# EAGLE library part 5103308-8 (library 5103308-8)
HEADER, 2.54MM, 40WAY
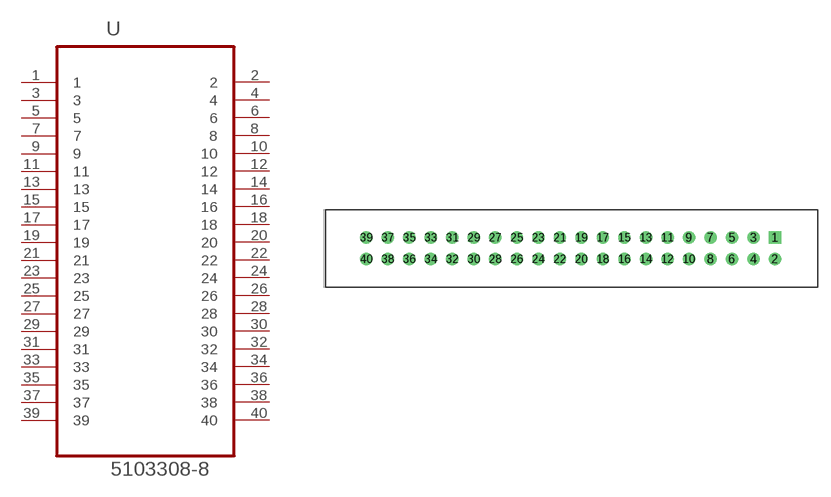
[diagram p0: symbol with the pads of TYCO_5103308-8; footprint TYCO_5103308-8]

Designator prefix U

## 5103308-8 (Centerline_Pitch: 2.54 mm[.1 in]; Comment: 5103308-8; Description: A/L LOW PRO HDR 40P VERT BLACK; Digi-Key_Part_Number: A33170-ND; Digi-Key_Purchase_URL: https://www.digikey.com/product-detail/en/te-connectivity-amp-connectors/5103308-8/A33170-ND/1114908?utm_source=snapeda&utm_medium=aggregator&utm_campaign=symbol; EU_RoHS_Compliance: Compliant; MF: TE Connectivity; MP: 5103308-8; Number_of_Positions: 40; Package: None; Product_Type: Connector; TE_purchase_URL: https://www.te.com/usa-en/product-5103308-8.html?te_bu=Cor&te_type=disp&te_campaign=seda_glo_cor-seda-global-disp-prtnr-fy19-seda-model-bom-cta_sma-317_1&elqCampaignId=32493)  [TYCO_5103308-8]
1  1  pas
2  2  pas
3  3  pas
4  4  pas
5  5  pas
6  6  pas
7  7  pas
8  8  pas
9  9  pas
10  10  pas
11  11  pas
12  12  pas
13  13  pas
14  14  pas
15  15  pas
16  16  pas
17  17  pas
18  18  pas
19  19  pas
20  20  pas
21  21  pas
22  22  pas
23  23  pas
24  24  pas
25  25  pas
26  26  pas
27  27  pas
28  28  pas
29  29  pas
30  30  pas
31  31  pas
32  32  pas
33  33  pas
34  34  pas
35  35  pas
36  36  pas
37  37  pas
38  38  pas
39  39  pas
40  40  pas

## Footprint TYCO_5103308-8 (pad centres in mm)
drill 0.965 square: 1 0,2.54
drill 0.965: 2 0,0; 3 -2.54,2.54; 4 -2.54,0; 5 -5.08,2.54; 6 -5.08,0; 7 -7.62,2.54; 8 -7.62,0; 9 -10.16,2.54; 10 -10.16,0; 11 -12.7,2.54; 12 -12.7,0; 13 -15.24,2.54; 14 -15.24,0; 15 -17.78,2.54; 16 -17.78,0; 17 -20.32,2.54; 18 -20.32,0; 19 -22.86,2.54; 20 -22.86,0; 21 -25.4,2.54; 22 -25.4,0; 23 -27.94,2.54; 24 -27.94,0; 25 -30.48,2.54; 26 -30.48,0; 27 -33.02,2.54; 28 -33.02,0; 29 -35.56,2.54; 30 -35.56,0; 31 -38.1,2.54; 32 -38.1,0; 33 -40.64,2.54; 34 -40.64,0; 35 -43.18,2.54; 36 -43.18,0; 37 -45.72,2.54; 38 -45.72,0; 39 -48.26,2.54; 40 -48.26,0

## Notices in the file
This work is licensed under a Creative Commons Attribution-ShareAlike 4.0 International License (CC BY-SA) with Design Exception 1.0
